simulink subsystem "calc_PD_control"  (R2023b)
settings: Solver=VariableStepAuto  StartTime=0.0  StopTime=10.0  RelTol=1e-3

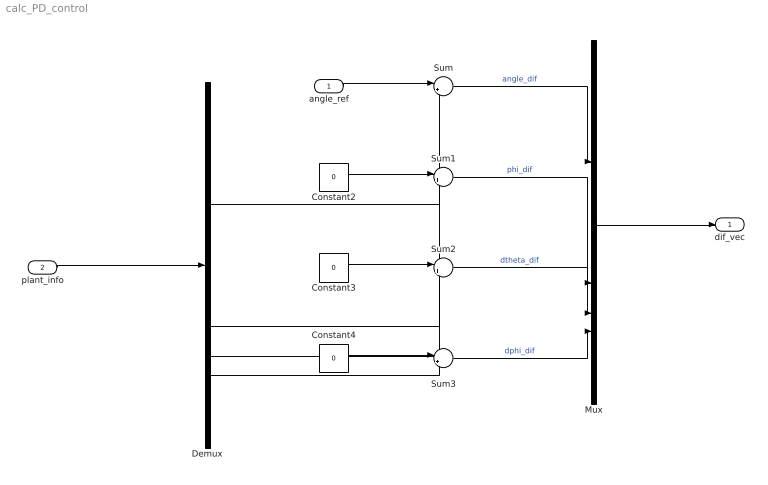
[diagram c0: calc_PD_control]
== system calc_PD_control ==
  angle_ref : Inport
  plant_info : Inport  Port=2  OutDataTypeStr=single  PortDimensions=4
  Constant2 : Constant  Value=0  OutDataTypeStr=single
  Constant3 : Constant  Value=0  OutDataTypeStr=single
  Constant4 : Constant  Value=0  OutDataTypeStr=single
  Demux : Demux
  Mux : Mux
  Sum{,1..3} (4 alike) : Sum  Inputs=|+-
  dif_vec : Outport
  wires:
  Constant3/1 -> Sum2/1
  angle_ref/1 -> Sum/1
  Demux/4 -> Sum3/2
  Demux/1 -> Sum/2
  Constant4/1 -> Sum3/1
  Constant2/1 -> Sum1/1
  Sum3/1 -> Mux/4  "dphi_dif"
  Sum/1 -> Mux/1  "angle_dif"
  plant_info/1 -> Demux/1
  Sum1/1 -> Mux/2  "phi_dif"
  Sum2/1 -> Mux/3  "dtheta_dif"
  Demux/3 -> Sum2/2
  Mux/1 -> dif_vec/1
  Demux/2 -> Sum1/2
